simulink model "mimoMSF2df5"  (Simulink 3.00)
settings: Solver=ode45  StartTime=0.0  StopTime=50.0  RelTol=1e-3
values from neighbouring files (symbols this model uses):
  Disturb = Setpoint    [mimo_MSF1DF_sim.m]    (also in mimo_MSF2DF_sim.m)
  K = 1/kpd    [imc2pseucon.m]    (also in imc2pseudo.m)
  Satlb = temp1    [cback.m]    (also in imcmenu.m = str2num(satlbs))
  Satub = temp1    [cback.m]    (also in imcmenu.m = str2num(satubs))
  Setpoint = zeros(1,n)    [mimo_MSF1DF_sim.m]    (also in mimo_MSF2DF_sim.m)
undefined symbols (not defined in the file or in its folder): Ds, input_delay, Kdelay, Ksp, T
libraries: simulink3 x28, MIMO_lib x28

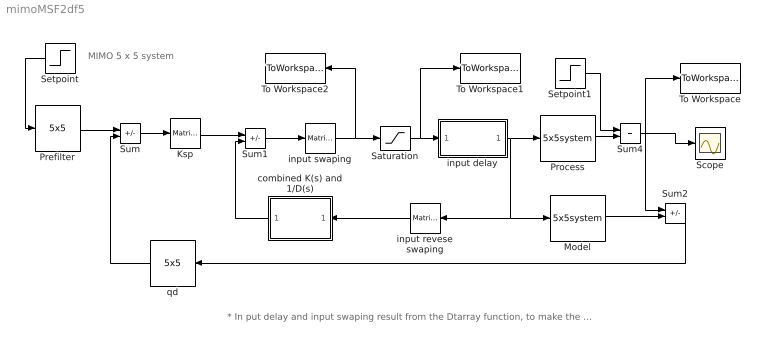
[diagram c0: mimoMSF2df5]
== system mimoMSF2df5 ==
  note: * In put delay and input swaping result from the Dtarray function, to make the system be able to be decoupled.
  note: MIMO 5 x 5 system
  Ksp : simulink3/Math/Matrix Gain  K=Ksp
  Model : MIMO_lib/5x5system  num=Mnum  den=Mden  dead=Mdead
  Prefilter : MIMO_lib/5x5  num=prefilnum  den=prefilden
  Process : MIMO_lib/5x5system  num=Pnum  den=Pden  dead=Pdead
  Saturation : Saturate  UpperLimit=Satub  LowerLimit=Satlb
  Scope : Scope
  Setpoint : Step  Orientation=left  Time=0  Before=0  After=[Setpoint]  SampleTime=0
  Setpoint1 : Step  Time=0  Before=0  After=[Disturb]  SampleTime=0
  Sum : Sum  Inputs=+-  SaturateOnIntegerOverflow=on
  Sum1 : Sum  Inputs=+-  SaturateOnIntegerOverflow=on
  Sum2 : Sum  Inputs=+-  SaturateOnIntegerOverflow=on
  Sum4 : Sum  Inputs=++  SaturateOnIntegerOverflow=on
  To Workspace : ToWorkspace  VariableName=yout  SampleTime=0  SaveFormat=Matrix
  To Workspace1 : ToWorkspace  VariableName=sat_effort  SampleTime=0  SaveFormat=Matrix
  To Workspace2 : ToWorkspace  VariableName=unsat_effort  SampleTime=0  SaveFormat=Matrix
  combined K(s) and 1/D(s) : Subsystem  Orientation=left  mask(ksds){Ksp=Ksp, Ds=Ds, Kdelay=Kdelay, K=K}
      mask prompts: Ds "D(s)"; Kdelay "Bdelay"; K "B*(s)"
  input delay : Subsystem  mask(input delay){input_delay=input_delay}
      mask prompts: input_delay "Input Delay (vector)"
  input revese swaping : simulink3/Math/Matrix Gain  Orientation=left  K=T
  input swaping : simulink3/Math/Matrix Gain  K=inv(T)
  qd : MIMO_lib/5x5  Orientation=left  num=qdnum  den=qdden
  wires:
  Ksp/1 -> Sum1/1
  combined K(s) and 1/D(s)/1(Out1) -> Sum1/2
  Sum/1 -> Ksp/1
  input revese swaping/1 -> combined K(s) and 1/D(s)/1(In1)
  Model/1 -> Sum2/2
  Process/1 -> Sum4/2
  Setpoint1/1 -> Sum4/1
  Sum4/1 -> Sum2/1, To Workspace/1, Scope/1
  input swaping/1 -> Saturation/1, To Workspace2/1
  Sum1/1 -> input swaping/1
  input delay/1(Out1) -> Process/1, Model/1, input revese swaping/1
  Saturation/1 -> input delay/1(In1), To Workspace1/1
  Prefilter/1 -> Sum/1
  Setpoint/1 -> Prefilter/1
  Sum2/1 -> qd/1
  qd/1 -> Sum/2

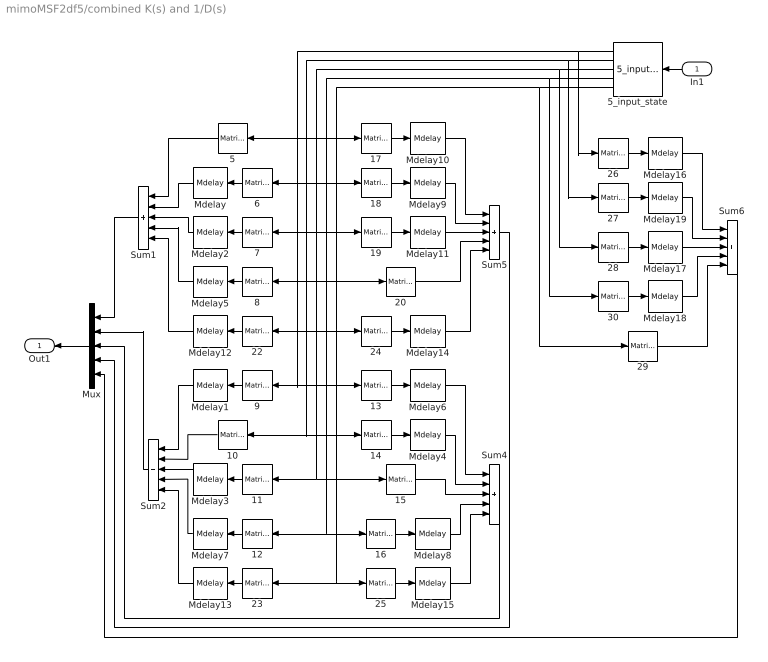
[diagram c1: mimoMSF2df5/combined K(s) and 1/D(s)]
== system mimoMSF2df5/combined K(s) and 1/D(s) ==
  In1 : Inport  Orientation=left  Port=1  PortWidth=-1  SampleTime=-1  DataType=auto
  10 : simulink3/Math/Matrix Gain  Orientation=left  K="[zeros(1,length(Ds{2})-length(K{2,2}))  K{2,2}]"
  11 : simulink3/Math/Matrix Gain  Orientation=left  K="[zeros(1,length(Ds{3})-length(K{2,3}))  K{2,3}]"
  12 : simulink3/Math/Matrix Gain  Orientation=left  K="[zeros(1,length(Ds{4})-length(K{2,4}))  K{2,4}]"
  13 : simulink3/Math/Matrix Gain  K="[zeros(1,length(Ds{1})-length(K{3,1}))  K{3,1}]"
  14 : simulink3/Math/Matrix Gain  K="[zeros(1,length(Ds{2})-length(K{3,2}))  K{3,2}]"
  15 : simulink3/Math/Matrix Gain  K="[zeros(1,length(Ds{3})-length(K{3,3}))  K{3,3}]"
  16 : simulink3/Math/Matrix Gain  K="[zeros(1,length(Ds{4})-length(K{3,4}))  K{3,4}]"
  17 : simulink3/Math/Matrix Gain  K="[zeros(1,length(Ds{1})-length(K{4,1}))  K{4,1}]"
  18 : simulink3/Math/Matrix Gain  K="[zeros(1,length(Ds{2})-length(K{4,2}))  K{4,2}]"
  19 : simulink3/Math/Matrix Gain  K="[zeros(1,length(Ds{3})-length(K{4,3}))  K{4,3}]"
  20 : simulink3/Math/Matrix Gain  K="[zeros(1,length(Ds{4})-length(K{4,4}))  K{4,4}]"
  22 : simulink3/Math/Matrix Gain  Orientation=left  K="[zeros(1,length(Ds{4})-length(K{1,4}))  K{1,4}]"
  23 : simulink3/Math/Matrix Gain  Orientation=left  K="[zeros(1,length(Ds{4})-length(K{2,4}))  K{2,4}]"
  24 : simulink3/Math/Matrix Gain  K="[zeros(1,length(Ds{5})-length(K{4,5}))  K{4,5}]"
  25 : simulink3/Math/Matrix Gain  K="[zeros(1,length(Ds{5})-length(K{3,5}))  K{3,5}]"
  26 : simulink3/Math/Matrix Gain  K="[zeros(1,length(Ds{1})-length(K{5,1}))  K{5,1}]"
  27 : simulink3/Math/Matrix Gain  K="[zeros(1,length(Ds{2})-length(K{5,2}))  K{5,2}]"
  28 : simulink3/Math/Matrix Gain  K="[zeros(1,length(Ds{3})-length(K{5,3}))  K{5,3}]"
  29 : simulink3/Math/Matrix Gain  K="[zeros(1,length(Ds{5})-length(K{5,5}))  K{5,5}]"
  30 : simulink3/Math/Matrix Gain  K="[zeros(1,length(Ds{5})-length(K{5,4}))  K{5,4}]"
  5 : simulink3/Math/Matrix Gain  Orientation=left  K="[zeros(1,length(Ds{1})-length(K{1,1}))  K{1,1}]"
  5_input_state : MIMO_lib/5_input_state  Orientation=left
  6 : simulink3/Math/Matrix Gain  Orientation=left  K=[zeros(1,length(Ds{2})-length(K{1,2})) K{1,2}]
  7 : simulink3/Math/Matrix Gain  Orientation=left  K="[zeros(1,length(Ds{3})-length(K{1,3}))  K{1,3}]"
  8 : simulink3/Math/Matrix Gain  Orientation=left  K="[zeros(1,length(Ds{4})-length(K{1,4}))  K{1,4}]"
  9 : simulink3/Math/Matrix Gain  Orientation=left  K="[zeros(1,length(Ds{1})-length(K{2,1}))  K{2,1}]"
  Mdelay : MIMO_lib/Mdelay  Orientation=left  Mdelay=Kdelay(1,2)
  Mdelay1 : MIMO_lib/Mdelay  Orientation=left  Mdelay=Kdelay(2,1)
  Mdelay10 : MIMO_lib/Mdelay  Mdelay=Kdelay(4,1)
  Mdelay11 : MIMO_lib/Mdelay  Mdelay=Kdelay(4,3)
  Mdelay12 : MIMO_lib/Mdelay  Orientation=left  Mdelay=Kdelay(1,4)
  Mdelay13 : MIMO_lib/Mdelay  Orientation=left  Mdelay=Kdelay(2,4)
  Mdelay14 : MIMO_lib/Mdelay  Mdelay=Kdelay(4,5)
  Mdelay15 : MIMO_lib/Mdelay  Mdelay=Kdelay(3,5)
  Mdelay16 : MIMO_lib/Mdelay  Mdelay=Kdelay(4,1)
  Mdelay17 : MIMO_lib/Mdelay  Mdelay=Kdelay(5,3)
  Mdelay18 : MIMO_lib/Mdelay  Mdelay=Kdelay(5,4)
  Mdelay19 : MIMO_lib/Mdelay  Mdelay=Kdelay(5,2)
  Mdelay2 : MIMO_lib/Mdelay  Orientation=left  Mdelay=Kdelay(1,3)
  Mdelay3 : MIMO_lib/Mdelay  Orientation=left  Mdelay=Kdelay(2,3)
  Mdelay4 : MIMO_lib/Mdelay  Mdelay=Kdelay(3,2)
  Mdelay5 : MIMO_lib/Mdelay  Orientation=left  Mdelay=Kdelay(1,4)
  Mdelay6 : MIMO_lib/Mdelay  Mdelay=Kdelay(3,1)
  Mdelay7 : MIMO_lib/Mdelay  Orientation=left  Mdelay=Kdelay(2,4)
  Mdelay8 : MIMO_lib/Mdelay  Mdelay=Kdelay(3,4)
  Mdelay9 : MIMO_lib/Mdelay  Mdelay=Kdelay(4,2)
  Mux : Mux  Orientation=left  Inputs=5
  Sum1 : Sum  Orientation=left  Inputs=+++++  SaturateOnIntegerOverflow=on
  Sum2 : Sum  Orientation=left  Inputs=+++++  SaturateOnIntegerOverflow=on
  Sum4 : Sum  Inputs=+++++  SaturateOnIntegerOverflow=on
  Sum5 : Sum  Inputs=+++++  SaturateOnIntegerOverflow=on
  Sum6 : Sum  Inputs=+++++  SaturateOnIntegerOverflow=on
  Out1 : Outport  Orientation=left  Port=1
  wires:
  Sum2/1 -> Mux/2
  Mux/1 -> Out1/1
  Sum1/1 -> Mux/1
  5/1 -> Sum1/1
  Mdelay/1 -> Sum1/2
  Mdelay2/1 -> Sum1/3
  6/1 -> Mdelay/1
  7/1 -> Mdelay2/1
  8/1 -> Mdelay5/1
  Mdelay5/1 -> Sum1/4
  Sum4/1 -> Mux/3
  Mdelay10/1 -> Sum5/1
  17/1 -> Mdelay10/1
  18/1 -> Mdelay9/1
  Mdelay9/1 -> Sum5/2
  19/1 -> Mdelay11/1
  Mdelay11/1 -> Sum5/3
  20/1 -> Sum5/4
  Sum5/1 -> Mux/4
  22/1 -> Mdelay12/1
  9/1 -> Mdelay1/1
  Mdelay1/1 -> Sum2/1
  10/1 -> Sum2/2
  11/1 -> Mdelay3/1
  Mdelay3/1 -> Sum2/3
  12/1 -> Mdelay7/1
  Mdelay7/1 -> Sum2/4
  Mdelay12/1 -> Sum1/5
  23/1 -> Mdelay13/1
  Mdelay13/1 -> Sum2/5
  Mdelay6/1 -> Sum4/1
  15/1 -> Sum4/3
  13/1 -> Mdelay6/1
  14/1 -> Mdelay4/1
  16/1 -> Mdelay8/1
  Mdelay8/1 -> Sum4/4
  Mdelay4/1 -> Sum4/2
  24/1 -> Mdelay14/1
  Mdelay14/1 -> Sum5/5
  25/1 -> Mdelay15/1
  Mdelay15/1 -> Sum4/5
  In1/1 -> 5_input_state/1
  Mdelay16/1 -> Sum6/1
  26/1 -> Mdelay16/1
  27/1 -> Mdelay19/1
  Mdelay19/1 -> Sum6/2
  28/1 -> Mdelay17/1
  Mdelay17/1 -> Sum6/3
  30/1 -> Mdelay18/1
  5_input_state/1 -> 26/1, 5/1, 17/1, 9/1, 13/1
  5_input_state/2 -> 27/1, 6/1, 18/1, 10/1, 14/1
  5_input_state/3 -> 28/1, 7/1, 19/1, 11/1, 15/1
  5_input_state/4 -> 30/1, 8/1, 20/1, 12/1, 16/1
  5_input_state/5 -> 29/1, 22/1, 24/1, 23/1, 25/1
  Mdelay18/1 -> Sum6/4
  29/1 -> Sum6/5
  Sum6/1 -> Mux/5

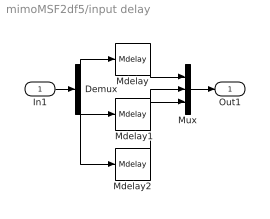
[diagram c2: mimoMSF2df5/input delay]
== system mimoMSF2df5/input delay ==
  In1 : Inport  Port=1  PortWidth=-1  SampleTime=-1  DataType=auto
  Demux : Demux  Outputs=3
  Mdelay : MIMO_lib/Mdelay  Mdelay=input_delay(1)
  Mdelay1 : MIMO_lib/Mdelay  Mdelay=input_delay(2)
  Mdelay2 : MIMO_lib/Mdelay  Mdelay=input_delay(3)
  Mux : Mux  Inputs=3
  Out1 : Outport  Port=1
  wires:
  Mux/1 -> Out1/1
  In1/1 -> Demux/1
  Demux/1 -> Mdelay/1
  Demux/2 -> Mdelay1/1
  Mdelay/1 -> Mux/1
  Mdelay1/1 -> Mux/2
  Demux/3 -> Mdelay2/1
  Mdelay2/1 -> Mux/3
